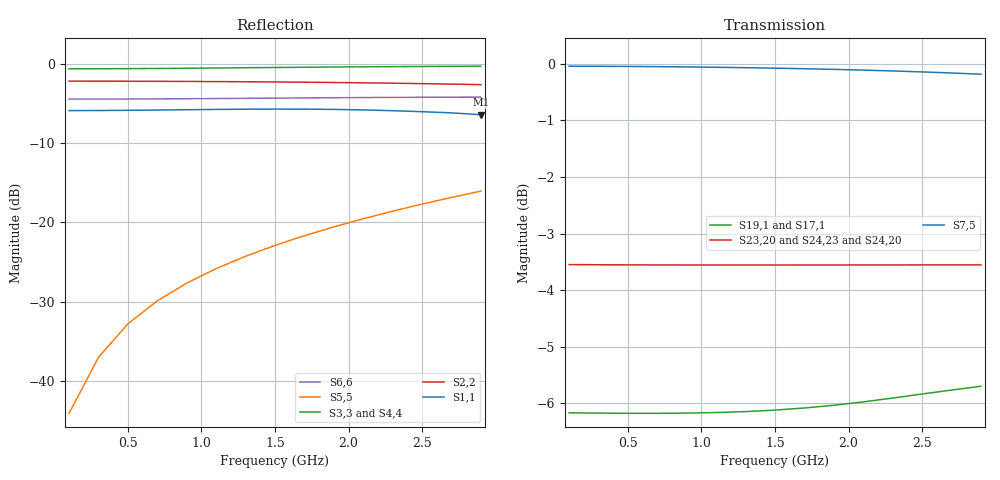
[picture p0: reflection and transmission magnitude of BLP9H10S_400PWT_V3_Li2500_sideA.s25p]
! Touchstone file from project OMP_EMMA_Packages_wk1818_Final
! Exported from HFSS 2018.0.0
! Variables:
!  AirBoxH = 25000um
!  AirBoxL = 30000um
!  AirBoxW = 55000um
!  PCB_H = 760um
# GHZ S MA R 50.000000
! Terminal data exported
! Port[1] = GT
! Port[2] = DT
! Port[3] = GD
! Port[4] = DD
! Port[5] = Box3_T1
! Port[6] = Box3_1_T1
! Port[7] = Rectangle2_T1
! Port[8] = Rectangle3_T1
! Port[9] = P1_BWT2_Rect_T1
! Port[10] = P2_BWT2_Rect_T1
! Port[11] = P3_BWT2_Rect_T1
! Port[12] = P4_BWT2_Rect_T1
! Port[13] = P5_BWT2_Rect_T1
! Port[14] = P6_BWT2_Rect_T1
! Port[15] = P7_BWT2_Rect_T1
! Port[16] = P8_BWT2_Rect_T1
! Port[17] = P9_BWT3_5_Rect_T1
! Port[18] = P10_BWT10_12_Rect_T1
! Port[19] = P11_BWT7_Rect_T1
! Port[20] = P12_BWT12_Rect_T1
! Port[21] = P13_BWT11_Rect_T1
! Port[22] = P14_BWT12_Rect_T1
! Port[23] = P15_BWT11_Rect_T1
! Port[24] = P16_BWT12_Rect_T1
! Port[25] = P17_BWT6_8_Rect_T1
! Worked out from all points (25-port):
!   15 points, 100 MHz to 2.9 GHz, reference per port
!   strongest paths, dB at 100 MHz, 700 MHz, 1.5 GHz, 2.3 GHz, 2.9 GHz:
!     S7,5: 0.0, 0.0, -0.1, -0.1, -0.2
!     S23,20: -3.5, -3.6, -3.6, -3.6, -3.6
!     S24,23: -3.5, -3.5, -3.6, -3.6, -3.7
!     S24,20: -3.6, -3.6, -3.6, -3.7, -3.8
!     S19,1: -6.2, -6.2, -6.1, -5.9, -5.7
!     S17,1: -6.2, -6.2, -6.3, -6.2, -5.8
!   lowest |S11| = -6.4 dB at 2.9 GHz (marker M1), VSWR 2.83
!   |S11| at or under -10 dB: nowhere
